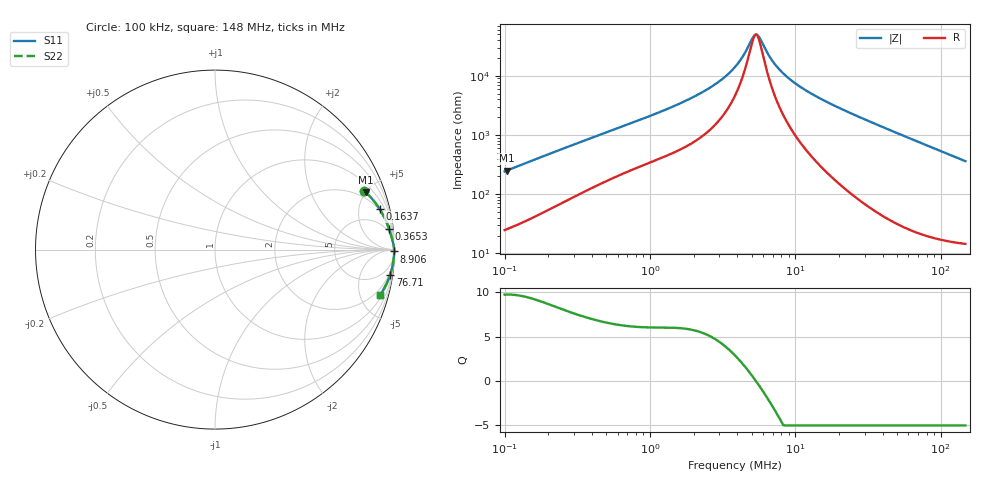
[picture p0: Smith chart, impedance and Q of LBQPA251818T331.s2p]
! LBQPA251818T331  S-PARAMETER MODEL  ( General Type )
! Model Generated by TAIYO YUDEN Corporation (http://www.ty-top.com)
! Version 1.0
! TAIYO YUDEN Control No. 191025NI43SB-FBB
! Copyright(c) 2019 TAIYO YUDEN CO.,LTD. All Rights Reserved.
! Product Description (link to TY-COMPAS)
! https://ds.yuden.co.jp/TYCOMPAS/or/detail?pn=LBQPA251818T331K&u=M
! Products Name : Inductors
! Characteristics :
!  Inductance : 330 uH , SRF(min) : 4.5 MHz , DC Resistance(max) : 15.99 Ohm
!  Rated Current : Saturation :100 mA , Temp Rise : 65 mA (20 degC)
!  Case Size : 2.5 x 1.8 / 0.098 x 0.071 [mm/inch] , Thickness : 1.8 / 0.071 [mm/inch]
!  (Conditions: Temperature = 25 degC , DC Bias Current/Voltage = 0A / 0V)
! External Node Assignments :
!  1  o---GGG---o  2
! GND o---------o GND
! Frequency Range : 0.1MHz  -  147.97148MHz  [ 402 STEP ]
# MHz S RI R 50
! Freq[MHz].  S11 Real  S11 Imag  S21 Real  S21 Imag  S12 Real  S12 Imag  S22 Real  S22 Imag
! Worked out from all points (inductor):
!   401 points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, 100 kHz to 148 MHz, reference 50 ohm
!   read as one part in series: L = 381 uH near 103.7 kHz
!   highest Q = 9.73 at 103.7 kHz (marker M1), where L = 383 uH
!   self-resonance near 5.343 MHz
!   S11 on the Smith chart (normalised r, x): 100 kHz: 1.50, +4.82; 163.7 kHz: 1.85, +7.76; 365.3 kHz: 3, +16; 8.906 MHz: open; 76.71 MHz: 1, -14; 148 MHz: 1.29, -7.22
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0.1  0.8305 0.3273  0.1695 -0.3273  0.1695 -0.3273  0.8305 0.3273
0.103717  0.8392 0.3196  0.1608 -0.3196  0.1608 -0.3196  0.8392 0.3196
0.163677  0.9166 0.2272  0.0834 -0.2272  0.0834 -0.2272  0.9166 0.2272
0.339629  0.9675 0.1217  0.0325 -0.1217  0.0325 -0.1217  0.9675 0.1217
0.365348  0.9701 0.1141  0.0299 -0.1141  0.0299 -0.1141  0.9701 0.1141
1.153479  0.9916 0.0404  0.0084 -0.0404  0.0084 -0.0404  0.9916 0.0404
1.787394  0.995 0.0254  0.00499 -0.0254  0.00499 -0.0254  0.995 0.0254
2.482438  0.9965 0.0165  0.00346 -0.0165  0.00346 -0.0165  0.9965 0.0165
3.205048  0.9973 0.0106  0.00272 -0.0106  0.00272 -0.0106  0.9973 0.0106
3.917549  0.9977 0.00631  0.00234 -0.00631  0.00234 -0.00631  0.9977 0.00631
4.370862  0.9978 0.00408  0.00219 -0.00408  0.00219 -0.00408  0.9978 0.00408
5.151054  0.998 0.000793  0.00203 -0.000793  0.00203 -0.000793  0.998 0.000793
5.440922  0.998 -0.000296  0.00199 0.000296  0.00199 0.000296  0.998 -0.000296
5.747101  0.998 -0.00139  0.00195 0.00139  0.00195 0.00139  0.998 -0.00139
6.412117  0.9981 -0.00359  0.00191 0.00359  0.00191 0.00359  0.9981 -0.00359
7.024715  0.9981 -0.00546  0.00188 0.00546  0.00188 0.00546  0.9981 -0.00546
8.905524  0.9981 -0.0106  0.0019 0.0106  0.0019 0.0106  0.9981 -0.0106
13.06453  0.9978 -0.0203  0.00216 0.0203  0.00216 0.0203  0.9978 -0.0203
20.99691  0.9968 -0.0366  0.00317 0.0366  0.00317 0.0366  0.9968 -0.0366
44.37094  0.9909 -0.081  0.00908 0.081  0.00908 0.081  0.9909 -0.081
76.71177  0.9761 -0.139  0.0239 0.139  0.0239 0.139  0.9761 -0.139
147.9715  0.9202 -0.2517  0.0798 0.2517  0.0798 0.2517  0.9202 -0.2517
